ORGANIZATION_BLOCK MAIN:OB1
TITLE= Ciclo elettropneumatico (A+ B+)/A-/B-
// Simulatore: 05
// Versione: 1.0
// Data: 28/02/2002
//------------ DESCRIZIONE DEL CONTROLLO ---------------------
// L'esempio utilizza due cilindri (A e B) a doppio effetto e due
// elettrovalvole 5/2 bistabili (1V1 e 2V1).
// Una valvola 3/2 monostabile 0V permette la distribuzione dell'aria al
// circuito.
// Sulla mandata di ciascun cilindro sono preseti degli strozzatori
// unidirezionali che permettono di regolare separatamente la velocità
// delle singole corse dei pistoni.
// Il ciclo continuo inizia con la pressione del pulsante SB1 e potrà
// essere interrotto mediante il pulsante di Stop SB3.
// Il pulsante SB2 permette con la sua pressione di eseguire un ciclo
// singolo.
// Agli ingressi del PLC vengono collegati:
// - il selettore SA per il comando dell'aria compressa;
// - il pulsante di arresto ciclo SB3;
// - il pulsante di avvio ciclo automatico SB1;
// - Il pulsante di avvio del ciclo singolo SB2
// - i fine corsa magnetici a0, a1, b0, b1 per il controllo
//   della posizione dei pistoni dei cilindri A e B;
// Le segnalazioni sono affidate a due lampade HL1 e HL2 che indicano
// rispettivamente la presenza dell'aria e il ciclo in funzione.
//

BEGIN
NETWORK 1 //ON/OFF distributore Aria Compressa
//
LD I0.0 //S_SB6
= Q0.0 //E_0Y1
= Q0.5 //HL1

NETWORK 2 //Gestione Ciclo Automatico
//
LD I0.2 //P_SB1
O M0.0 //Ciclo ON
A I0.1 //P_SB3
= M0.0 //Ciclo ON
= Q0.6 //HL2

NETWORK 3 //Corsa  A+ B+
//
LD M0.0 //Ciclo ON
O I0.3 //P_SB2
A I0.6 //b0
= Q0.1 //E_1Y1
= Q0.3 //E_2Y1

NETWORK 4 //Corsa  A-
//
LD I0.5 //a1
O Q0.2 //E_1Y2
A I0.7 //b1
= Q0.2 //E_1Y2

NETWORK 5 //Corsa B-
//
LD I0.4 //a0
A Q0.2 //E_1Y2
= Q0.4 //E_2Y2

END_ORGANIZATION_BLOCK

